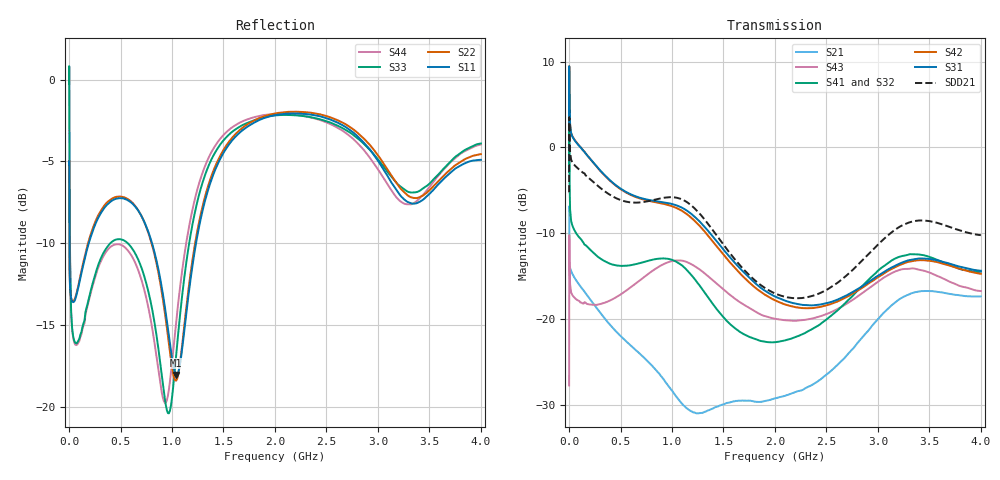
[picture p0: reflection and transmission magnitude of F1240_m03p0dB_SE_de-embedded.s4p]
! Integrated Device Technology
! Corporate Headquarters
! 6024 Silver Creek Valley Road
! San Jose, CA 95138  USA
! Phone:  1-408-284-8200
! Toll Free:  1-800-223-1366
! Webpage:  http://www.idt.com/
! Timing and RF Division
! 515 Groton Road, Suite 102
! Westford, MA 01886-6024
! Device:  F1240
! Description: Dual Intermediate Frequency Digital Variable Gain Amplifier
! Frequency:  10.0 -  500.00 MHz
! Package:  5x5 mm QFN Plastic Package: 32 pin
! Ports:  8 RF, 20 DC
!  Pin  1  = GA3 / Data  Pin 17  = RF OUT_B+
!  Pin  2  = GA4 / CLK  Pin 18  = RF OUT_B-
!  Pin  3  = GA5  Pin 19  = STBY_B
!  Pin  4  = VMODE  Pin 20  = Ground
!  Pin  5  = No Connect  Pin 21  = Ground
!  Pin  6  = GB5  Pin 22  = STB_A
!  Pin  7  = GB4  Pin 23  = RF OUT_A-  = Port 4
!  Pin  8  = GB3  Pin 24  = RF OUT_A+  = Port 3
!  Pin  9  = GB2  Pin 25  = GA0
!  Pin 10  = GB1  Pin 26  = ISET_A
!  Pin 11  = RF IN_B+  Pin 27  = VCC
!  Pin 12  = RF IN_B-  Pin 28  = Ground
!  Pin 13  = Ground  Pin 29  = RF IN_A-  = Port 2
!  Pin 14  = VCC  Pin 30  = RF IN_A+  = Port 1
!  Pin 15  = ISET_B  Pin 31  = GA1
!  Pin 16  = GB0  Pin 32  = GA2 / CSb
! Gain  = +19.5 dB
! State  = 1
! Voltage  = +5.00 V
! Current  = 85.292 mA (one channel only)
! Temperture  =  +25 C
! Test Date  =  2017-10-18
! Board  =  EB4031
! Data:  The device was measured on a custom evaluation board which has
!  individual transmission lines to the RF pins.  Data was collected
!  using a calibrated network analyzer.  The evaluation board was
!  de-embedded using Automatic Fixture Removal.
!  The reference plane is the edge of the package pin.
!  Only Channel A was measured.
!  This data is in single-ended operation.  If your needs are balanced
!  or differential S-parameters then this file needs to be used a
!  linear simulator.
! File Date:  2017-11-10  MJV
! Note:
!  Integrated Device Technology supplies this data as a sample of measured
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# Hz S dB R 100
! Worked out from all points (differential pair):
!   410 points, 500 kHz to 4 GHz, reference 100 ohm
!   strongest paths, dB at 500 kHz, 930 MHz, 1.96 GHz, 2.98 GHz, 4 GHz:
!     S31: 2.1, -6.4, -17.1, -15.1, -14.4
!     S42: 2.1, -6.6, -17.6, -15.3, -14.7
!     S41: -2.9, -13.0, -22.7, -14.6, -14.5
!     S32: -2.8, -13.1, -22.7, -15.0, -15.0
!     S43: -27.8, -13.5, -19.9, -15.8, -16.8
!     S21: -7.0, -27.3, -29.4, -20.3, -17.4
!   taken as a pair (ports 1,2 in; 3,4 out), SDD21 dB: -5.2, -5.9, -16.8, -11.6, -10.2
!   lowest |S11| = -18.0 dB at 1.04 GHz (marker M1), VSWR 1.29, Z = 78.8 - j7.43 ohm
!   |S11| at or under -10 dB: 3.259 MHz to 190.8 MHz (187.5 MHz wide, 193 % of centre); 806.3 MHz to 1.233 GHz (426.5 MHz wide, 41.8 % of centre)
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500000  -5.16 -5.6  -7.02 -5.8  -30.61 79.7  -35.82 77.9
        -7.04 -5.8  -5.15 -5.6  -35.80 76.9  -30.62 80.9
        2.05 -108.7  -2.83 -110.9  -0.24 0.5  -27.75 -40.3
        -2.86 -109.8  2.06 -107.5  -27.75 -40.3  -0.25 2.8
2000000  -7.27 -34.1  -9.72 -34.3  -21.48 27.7  -27.47 6.7
         -9.72 -34.3  -7.24 -34.2  -27.42 6.5  -21.47 28.0
         9.12 -177.5  3.61 164.1  -0.16 -49.9  -10.23 -138.8
         3.57 164.4  9.13 -177.2  -10.23 -138.9  -0.20 -49.5
4000000  -10.90 -32.5  -13.16 -24.4  -21.81 8.5  -30.74 -15.2
         -13.17 -24.4  -10.90 -32.8  -30.69 -15.4  -21.80 8.7
         5.92 159.7  -2.30 138.4  -4.65 -82.4  -12.53 177.2
         -2.35 138.6  5.92 159.9  -12.52 177.1  -4.70 -82.4
1.7e8  -10.48 -100.8  -17.15 -55.2  -24.21 -43.1  -35.72 -34.0
       -17.16 -55.2  -10.33 -102.2  -35.80 -33.6  -24.22 -43.4
       -0.84 116.8  -11.52 90.3  -13.93 -148.2  -18.25 110.4
       -11.50 90.1  -0.83 116.0  -18.22 110.0  -14.06 -148.2
1.04e9  -18.03 -158.3  -29.45 160.6  -24.12 151.5  -31.86 -167.9
        -29.04 160.4  -18.38 -154.7  -31.84 -163.0  -24.83 151.0
        -6.74 -92.1  -13.51 175.8  -16.84 -111.8  -13.35 -128.9
        -13.32 171.6  -7.05 -94.8  -13.18 -128.8  -14.80 -108.0
2.87e9  -3.90 95.7  -21.90 -28.5  -25.18 -152.0  -27.45 -136.5
        -21.85 -28.5  -3.64 96.8  -28.29 -124.2  -26.35 -146.5
        -16.02 -63.7  -16.27 -149.2  -3.97 100.8  -17.68 -84.5
        -15.90 -159.7  -16.19 -60.7  -16.81 -81.7  -4.35 93.7
4e9  -4.90 -141.7  -17.40 106.4  -23.64 -37.6  -24.75 -22.1
     -17.38 106.3  -4.55 -139.8  -25.70 -7.0  -25.35 -30.7
     -14.38 47.7  -14.98 -55.7  -3.90 -133.7  -18.41 65.7
     -14.49 -68.8  -14.74 53.7  -16.75 57.7  -3.96 -143.5
